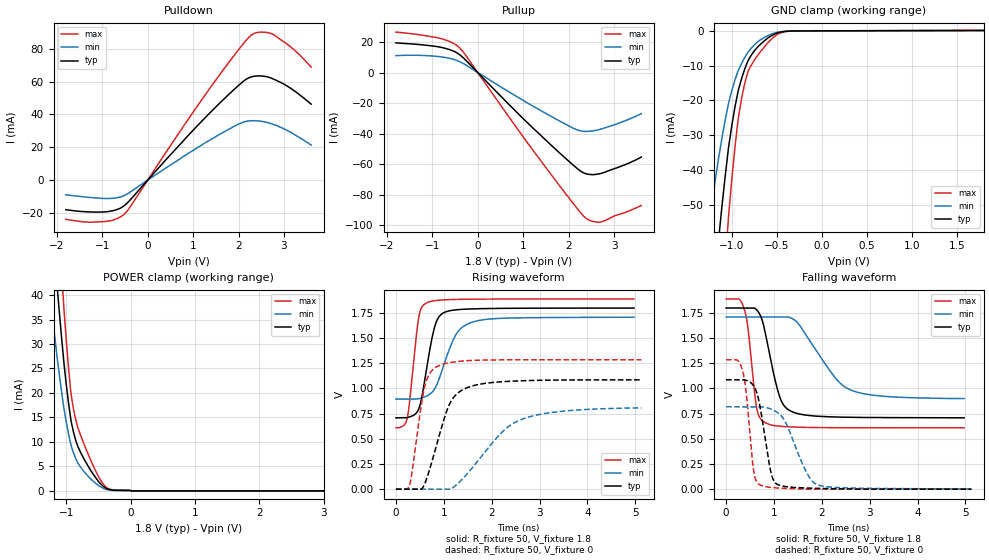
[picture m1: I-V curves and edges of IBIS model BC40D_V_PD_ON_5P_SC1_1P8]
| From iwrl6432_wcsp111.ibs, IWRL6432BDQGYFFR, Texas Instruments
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|   Model Cell BC40D_V_PD_ON_5P_SC1_1P8
|BC40D_V_PD_ON_5P_SC1_1P8
[Model]   BC40D_V_PD_ON_5P_SC1_1P8
Model_type   I/O
Polarity   Non-Inverting
Enable   Active-Low
Vinl =  0.63
Vinh =  1.17
Cref =  15pF
Rref =  100.0000M
Vref =  0V
Vmeas =  0.9
C_comp   2.233931p   2.204415p   2.290246p
|[Input load] weak_pd_on
|[Output drive] slow
|[supplytol] 5
|[temp] ind
[Model Spec]
Vinl   0.63   0.5985   0.6615
Vinh   1.17   1.1115   1.2285
[Temperature Range]   25   125   -40
[Voltage Range]   1.8   1.71   1.89
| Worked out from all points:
|   slope of the pulldown table from 0 to 0.27 V, typ, clamps not added: 32.2 ohm
|   slope of the pullup table from 0 to 0.27 V, typ, clamps not added: 32.6 ohm
|   GND clamp passes 1 mA (typ) near -0.53 V on its own axis
|   POWER clamp passes 1 mA (typ) near -0.43 V on its own axis
|   rising waveform, R_fixture 50, V_fixture 1.8: 20-80 % time 246ps typ, 396ps min, 169ps max; typ from 0.708 V to 1.8 V
|   rising waveform, R_fixture 50, V_fixture 0: 20-80 % time 429ps typ, 920ps min, 245ps max; typ from 0 V to 1.09 V
|   falling waveform, R_fixture 50, V_fixture 1.8: 20-80 % time 308ps typ, 717ps min, 171ps max; typ from 1.8 V to 0.708 V
|   falling waveform, R_fixture 50, V_fixture 0: 20-80 % time 226ps typ, 430ps min, 153ps max; typ from 1.08 V to 0 V
| Nom Voltages:
|   VDD=1.1, VDDS=1.8, VDDS18=1.8, ESD_BIASFET=0, VSS=0, VSSS=0
| Min Voltages:
|   VDD=1.045, VDDS=1.71, VDDS18=1.71, ESD_BIASFET=0, VSS=0, VSSS=0
| Max Voltages:
|   VDD=1.16, VDDS=1.89, VDDS18=1.89, ESD_BIASFET=0, VSS=0, VSSS=0
[POWER_clamp]
|   voltage   I(typ)   I(min)   I(max)
-1.8V     158.9mA    112.5mA    219.9mA
-1.255V   60.04mA    40.04mA    85.04mA
-1.145V   41.99mA    27.45mA    59.9mA
-1.109V   36.4mA     23.66mA    51.97mA
-1.073V   31.03mA    20.08mA    44.3mA
-1.036V   25.91mA    16.71mA    36.9mA
-927.3mV  14.27mA    9.301mA    19.77mA
-854.5mV  10.33mA    6.623mA    14.48mA
-454.5mV  1.273mA    746.6uA    1.931mA
-309.1mV  221.6uA    137.5uA    298.5uA
18.18mV   0A         0A         0A
3.6V      0A         0A         0A
[Pulldown]
|   voltage   I(typ)   I(min)   I(max)
-1.8V     -17.92mA   -8.85mA    -23.8mA
-1.309V   -19.26mA   -10.37mA   -25.5mA
-927.3mV  -19.22mA   -11.12mA   -25.08mA
-654.5mV  -17.65mA   -10.56mA   -23.13mA
-490.9mV  -14.97mA   -8.985mA   -20.05mA
1.364V    40.78mA    24.32mA    55.69mA
2.073V    59.4mA     35mA       81.9mA
2.291V    62.96mA    36.2mA     88.48mA
2.509V    63.41mA    35.84mA    90.12mA
2.782V    61.38mA    33.82mA    88.42mA
3.218V    54.59mA    28.02mA    79.45mA
3.6V      46.26mA    21.39mA    68.79mA
[Pullup]
|   voltage   I(typ)   I(min)   I(max)
-1.8V     19.42mA    11.07mA    26.5mA
-818.2mV  16.58mA    10.3mA     22.34mA
-545.5mV  14.19mA    8.748mA    19.29mA
-381.8mV  11.34mA    6.915mA    15.7mA
1.255V    -37.51mA   -22.64mA   -52.53mA
2.127V    -61.34mA   -36.82mA   -86.78mA
2.291V    -65.12mA   -38.38mA   -92.82mA
2.4V      -66.46mA   -38.59mA   -95.91mA
2.564V    -66.86mA   -38.08mA   -97.75mA
2.727V    -65.99mA   -36.9mA    -97.78mA
3.273V    -60.01mA   -31.26mA   -91.34mA
3.6V      -55.4mA    -26.98mA   -87.12mA
[GND_clamp]
|   voltage   I(typ)   I(min)   I(max)
-1.8V     -270.2mA   -170.2mA   -430.1mA
-1.255V   -91.66mA   -55.91mA   -148.4mA
-1.145V   -59.91mA   -36.45mA   -97.1mA
-1.109V   -50.48mA   -30.83mA   -81.56mA
-1.073V   -41.73mA   -25.65mA   -67.06mA
-1.036V   -33.67mA   -20.93mA   -53.6mA
-927.3mV  -17.08mA   -11.35mA   -25.06mA
-854.5mV  -10.88mA   -7.624mA   -14.94mA
-781.8mV  -6.944mA   -4.956mA   -9.81mA
-636.4mV  -2.852mA   -1.883mA   -4.567mA
-381.8mV  -107.5uA   -92.09uA   -158.2uA
1.8V      101.9uA    59.12uA    150.8uA
[Ramp]
| variable   typ   min   max
dV/dt_f 0.66096344/0.31032057n 0.49614538/0.73309515n 0.77261485/0.17237057n
dV/dt_r 0.65867605/0.43206823n 0.50260003/0.96153533n 0.77694652/0.24600924n
R_load = 50
[Rising Waveform]
R_fixture = 50
V_fixture = 1.8
V_fixture_min = 1.71
V_fixture_max = 1.89
|   time   V(typ)   V(min)   V(max)
0s        708.5mV    893.6mV    610.5mV
234.6ps   710.6mV    893.6mV    702.7mV
472.3ps   792.1mV    898mV      1.694V
530.6ps   888.5mV    905.2mV    1.798V
629.5ps   1.163V     922.2mV    1.847V
776.9ps   1.55V      974.4mV    1.869V
898.1ps   1.71V      1.09V      1.876V
1.247ns   1.78V      1.528V     1.884V
1.557ns   1.789V     1.652V     1.886V
4.974ns   1.798V     1.707V     1.887V
[Rising Waveform]
R_fixture = 50
V_fixture = 0
V_fixture_min = 0
V_fixture_max = 0
|   time   V(typ)   V(min)   V(max)
0s        0V         0V         0V
286.6ps   0V         0V         43.73mV
599.2ps   50.79mV    0V         1.013V
699.4ps   189mV      0V         1.144V
860.9ps   457.8mV    0V         1.218V
1.155ns   875.7mV    4.596mV    1.258V
1.568ns   1.021V     196.3mV    1.278V
2.232ns   1.067V     573.5mV    1.284V
2.671ns   1.077V     700.9mV    1.284V
5.128ns   1.086V     807mV      1.285V
[Falling Waveform]
R_fixture = 50
V_fixture = 1.8
V_fixture_min = 1.71
V_fixture_max = 1.89
|   time   V(typ)   V(min)   V(max)
0s        1.798V     1.708V     1.887V
275ps     1.798V     1.708V     1.887V
378.3ps   1.798V     1.708V     1.79V
458.2ps   1.798V     1.708V     1.598V
639.1ps   1.78V      1.708V     806.6mV
815.9ps   1.559V     1.708V     660.4mV
1.117ns   921.1mV    1.708V     624.7mV
1.373ns   769.9mV    1.695V     617.2mV
2.561ns   713.4mV    993.5mV    609.5mV
4.974ns   708mV      898.7mV    609.1mV
[Falling Waveform]
R_fixture = 50
V_fixture = 0
V_fixture_min = 0
V_fixture_max = 0
|   time   V(typ)   V(min)   V(max)
0s        1.085V     817.3mV    1.284V
342.4ps   1.085V     817.3mV    1.18V
418.5ps   1.081V     817.3mV    967.3mV
575.5ps   1.025V     817.3mV    189.7mV
702.7ps   837.4mV    817.3mV    43.74mV
935ps     172.5mV    795.6mV    17.12mV
1.095ns   42.28mV    753.2mV    11.14mV
1.696ns   10.81mV    154.4mV    0V
1.915ns   8.056mV    43.25mV    0V
5.128ns   0V         2.014mV    0V
